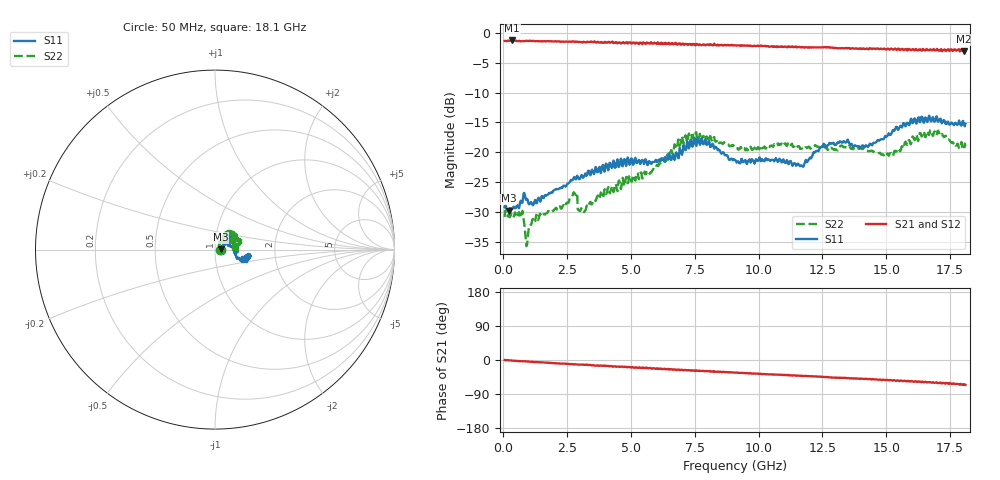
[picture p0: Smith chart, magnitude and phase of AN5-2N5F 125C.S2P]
! Network Analyzer HP8720D.06.14 Serial No. US36140669
! 12 Jan 2005  11:09:31
! Frequency  S11  S21  S12  S22
# HZ  S  DB R 50
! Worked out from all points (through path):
!   801 points, 50 MHz to 18.1 GHz, reference 50 ohm
!   highest |S21| = -1.23 dB at 343.3 MHz (marker M1); lowest = -3.1 dB at 18.03 GHz (marker M2)
!   group delay of S21, straight-line fit = 9.58 ps
!   lowest |S11| = -29.8 dB at 207.9 MHz (marker M3), VSWR 1.07, Z = 53.3 + j0.0681 ohm
!   |S11| at or under -10 dB: start of sweep to end of sweep
!   |S22| runs from -35.8 to -16.3 dB; largest |S21 - S12| = 0.029
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5e7  -29.21 -3.4  -1.30 0.0  -1.29 -0.6  -30.86 0.1
2.079375e8  -29.82 1.1  -1.27 -0.8  -1.27 -1.0  -30.59 -2.2
3.433125e8  -29.39 5.0  -1.23 -1.5  -1.26 -1.9  -30.60 -0.9
7.043125e8  -28.25 12.5  -1.36 -3.1  -1.35 -3.6  -30.54 6.5
9.299375e8  -27.84 7.5  -1.31 -4.1  -1.30 -4.1  -35.52 19.0
1.22325e9  -28.25 18.9  -1.36 -5.5  -1.33 -5.7  -31.82 31.1
2.351375e9  -25.61 28.5  -1.44 -9.7  -1.42 -10.0  -28.86 50.2
2.802625e9  -24.31 27.2  -1.49 -11.4  -1.46 -11.8  -27.05 55.3
3.073375e9  -23.82 33.0  -1.51 -12.5  -1.45 -12.9  -29.56 43.1
4.539938e9  -22.35 34.2  -1.55 -17.5  -1.64 -17.9  -24.75 51.2
6.074188e9  -21.52 33.3  -1.72 -23.9  -1.68 -23.7  -22.29 54.7
7.202312e9  -18.10 43.8  -1.87 -27.7  -1.78 -27.3  -18.30 44.3
7.969438e9  -18.75 43.7  -1.89 -29.0  -1.91 -29.9  -17.35 31.8
9.075e9  -21.30 33.0  -2.06 -33.3  -1.97 -33.7  -19.09 22.8
1.169225e10  -22.24 17.9  -2.35 -42.0  -2.29 -42.3  -19.36 26.0
1.209838e10  -20.69 9.3  -2.38 -42.8  -2.36 -43.3  -19.11 29.9
1.284294e10  -18.56 -4.1  -2.42 -46.2  -2.39 -46.5  -19.26 28.9
1.421925e10  -18.86 -9.4  -2.61 -49.7  -2.55 -50.1  -19.70 26.6
1.509919e10  -16.82 -19.9  -2.70 -53.8  -2.57 -53.6  -20.59 29.4
1.667856e10  -13.85 -10.9  -2.86 -58.4  -2.69 -59.1  -17.09 20.3
1.803231e10  -15.03 -20.7  -3.08 -64.4  -3.08 -66.0  -19.46 16.4
1.81e10  -15.25 -18.1  -2.96 -65.7  -2.95 -66.3  -19.00 8.5
